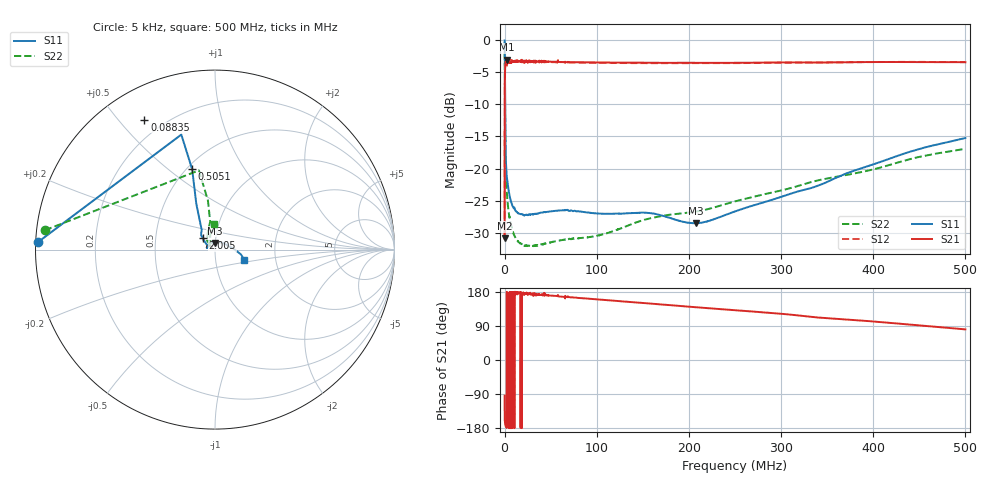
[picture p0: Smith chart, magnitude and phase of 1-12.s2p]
#  HZ  S  MA  R  50.00
! Rohde & Schwarz Vector Network Analyzer
! Rohde-Schwarz,ZNL6-2Port,1323001206101378,1.50.1.34-21.10.1.104
! Created: UTC 2/4/2024, 9:59:27 AM
! freq[Hz]  mag:S11  ang:S11  mag:S21  ang:S21  mag:S12  ang:S12  mag:S22  ang:S22
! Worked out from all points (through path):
!   6000 points, 5 kHz to 500 MHz, reference 50 ohm
!   highest |S21| = -3.11 dB at 2.505 MHz (marker M1); lowest = -30.8 dB at 5 kHz (marker M2)
!   lowest |S11| = -28.5 dB at 207.2 MHz (marker M3), VSWR 1.08, Z = 49.6 + j3.73 ohm
!   |S11| at or under -10 dB: 696.8 kHz to end of sweep
!   |S22| runs from -32.0 to -0.4 dB; largest |S21 - S12| = 0.2
!   S11 on the Smith chart (normalised r, x): 5 kHz: 0.01, +0.02; 88.35 kHz: 0.13, +0.59; 505.1 kHz: 0.53, +0.61; 2.005 MHz: 0.87, +0.11; 500 MHz: 1.38, -0.17
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5000  0.9862 177.5  0.02872 -93.8  0.02828 -93.5  0.9542 173.5
88346.39  0.8244 118.5  0.3009 -150.6  0.3348 -151.4  0.6149 112.7
505078.3  0.4652 105.9  0.5818 -167.5  0.6126 -173.0  0.2768 98.2
2005313  0.09251 136.3  0.6627 -176.8  0.664 -176.7  0.0726 131.7
2505392  0.08369 140.8  0.6989 -168.9  0.627 174.5  0.06256 131.0
2588738  0.08279 141.0  0.6953 -169.3  0.6337 174.9  0.0614 131.3
3005470  0.07933 140.9  0.6671 -175.6  0.674 -179.5  0.05662 132.4
3505548  0.07429 141.9  0.6635 -176.9  0.6807 -178.8  0.05224 133.4
6339326  0.05763 147.0  0.6645 -179.9  0.6902 179.5  0.03833 136.8
1.050665e7  0.04996 152.1  0.6772 175.6  0.6801 -178.9  0.03026 143.0
1.584081e7  0.04466 158.8  0.6801 177.1  0.6805 176.7  0.02667 148.4
3.284348e7  0.0444 164.2  0.6809 174.4  0.6728 171.0  0.0252 154.8
4.259501e7  0.04595 165.6  0.684 175.4  0.6681 166.1  0.02605 156.3
8.335139e7  0.04633 160.2  0.6678 163.2  0.6629 162.0  0.02894 153.7
1.08272e8  0.04454 147.8  0.6652 158.5  0.66 156.9  0.03109 143.5
1.666978e8  0.04395 123.4  0.6615 147.2  0.6571 145.7  0.04235 131.7
2.072041e8  0.03761 93.4  0.6615 139.3  0.6577 137.8  0.04635 123.9
2.500442e8  0.04651 62.3  0.6608 131.4  0.6579 129.1  0.05565 116.7
3.031358e8  0.06132 34.2  0.6664 121.3  0.6623 119.0  0.06844 112.5
3.333906e8  0.07091 19.6  0.6649 113.5  0.6643 113.2  0.07878 109.7
4.16737e8  0.1186 -3.2  0.671 98.2  0.6714 98.1  0.1062 100.2
5e8  0.1727 -20.1  0.668 80.8  0.6714 81.9  0.1424 92.0
